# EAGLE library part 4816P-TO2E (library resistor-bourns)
BOURNS RESISTOR NETWORK
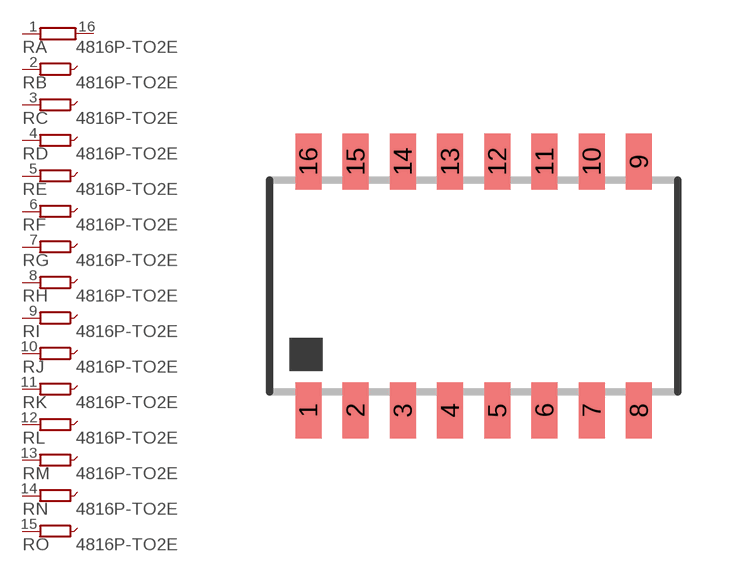
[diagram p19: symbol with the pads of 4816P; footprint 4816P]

Designator prefix R; gates A=R1NV B=R1NVXX C=R1NVXX D=R1NVXX E=R1NVXX F=R1NVXX G=R1NVXX H=R1NVXX I=R1NVXX J=R1NVXX K=R1NVXX L=R1NVXX M=R1NVXX N=R1NVXX O=R1NVXX

## 4816P-TO2E (OC_FARNELL: unknown; OC_NEWARK: unknown)  [4816P]
1  A:1  pas
2  B:1  pas
3  C:1  pas
4  D:1  pas
5  E:1  pas
6  F:1  pas
7  G:1  pas
8  H:1  pas
9  I:1  pas
10  J:1  pas
11  K:1  pas
12  L:1  pas
13  M:1  pas
14  N:1  pas
15  O:1  pas
16  A:2  pas

## Footprint 4816P (pad centres in mm)
BOURNS RESISTOR NETWORK
smd 0.7 x 1.5: 1 -4.445,-3.346; 2 -3.175,-3.346; 3 -1.905,-3.346; 4 -0.635,-3.346; 5 0.635,-3.346; 6 1.905,-3.346; 7 3.175,-3.346; 8 4.445,-3.346; 9 4.445,3.346; 10 3.175,3.346; 11 1.905,3.346; 12 0.635,3.346; 13 -0.635,3.346; 14 -1.905,3.346; 15 -3.175,3.346; 16 -4.445,3.346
